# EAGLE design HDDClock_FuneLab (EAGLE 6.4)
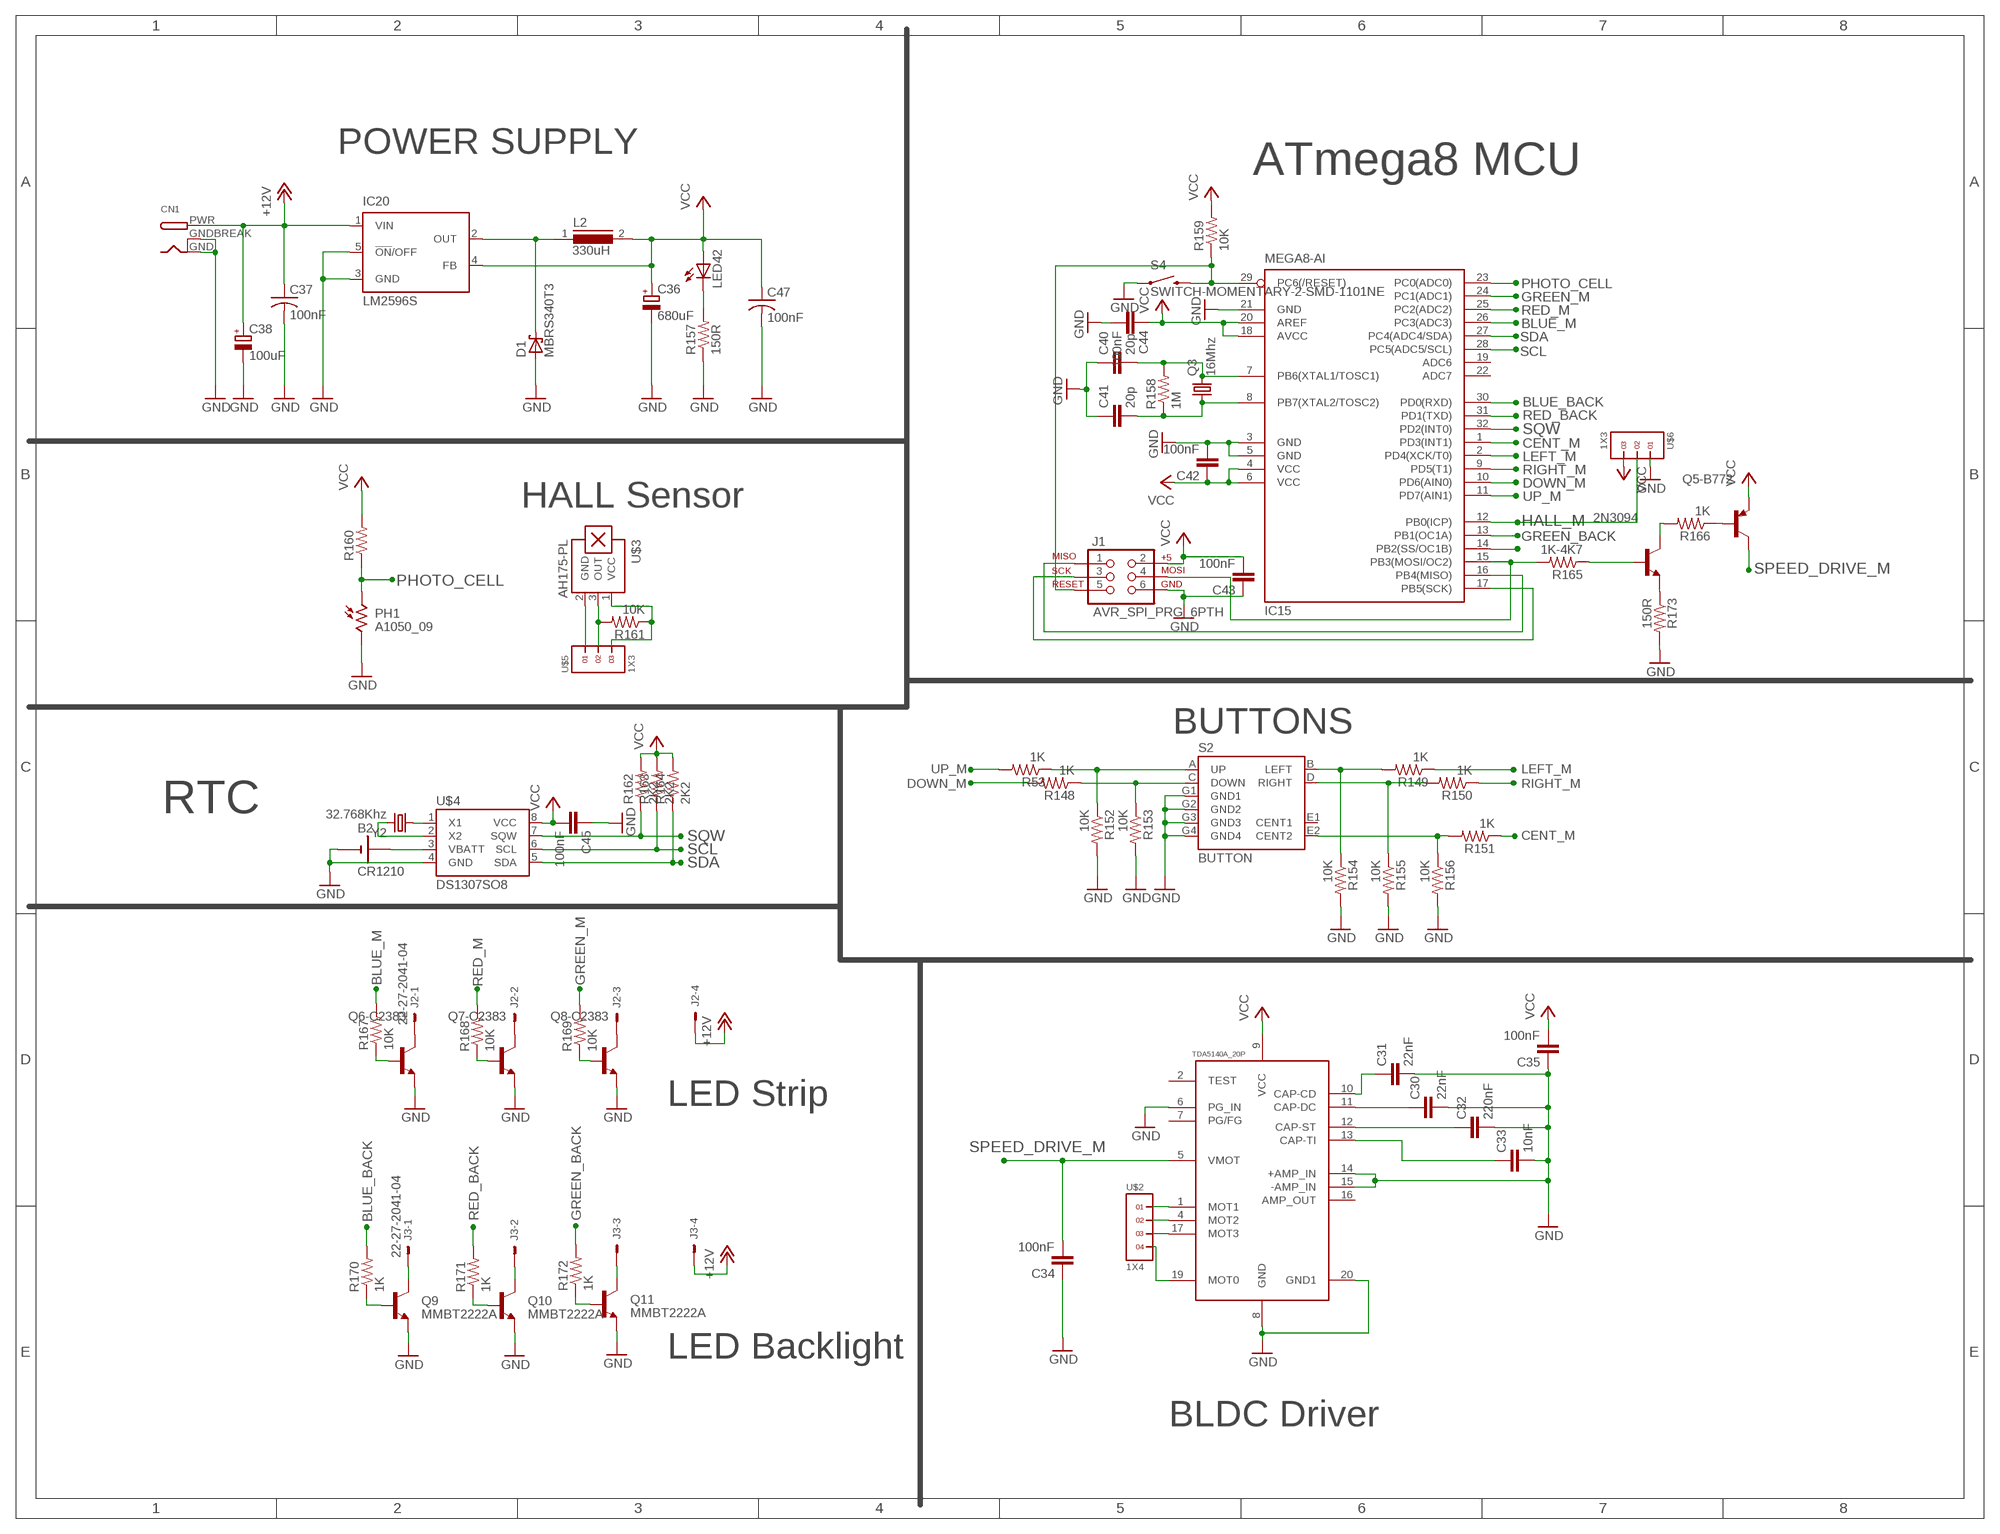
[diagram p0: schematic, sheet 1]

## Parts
2N3094  MMBT3904LT1-NPN-SOT23-BEC  [SOT23-BEC]
B2  CR1210  [CR1220_SMD]
C30  22nF  C-EUC0805K  [C0805K]
C31  22nF  C-EUC0805K  [C0805K]
C32  220nF  C-EUC0805K  [C0805K]
C33  10nF  C-EUC0805K  [C0805K]
C34  100nF  C5/2.5  [C5B2.5]
C35  100nF  C-EUC0603  [C0603]
C36  680uF  CPOL-EU153CLV-1012  [153CLV-1012]
C37  100nF  C-USC0805K  [C0805K]
C38  100uF  CPOL-EU153CLV-0605  [153CLV-0605]
C40  20p  C-EUC0603K  [C0603K]
C41  20p  C-EUC0603K  [C0603K]
C42  100nF  C-EUC0603K  [C0603K]
C43  100nF  C-EUC0603K  [C0603K]
C44  100nF  C-EUC0603K  [C0603K]
C45  100nF  C-EUC0603  [C0603]
C47  100nF  C-USC0805K  [C0805K]
CN1  DCBARRELPTH  [DCJACK_2MM_PTH]
D1  MBRS340T3  [SMC]
IC15  MEGA8-AI  [TQFP32-08]
IC20  LM2596S  [TO263-5]
J1  AVR_SPI_PRG_6PTH  [2X3]
J2  22-27-2041-04  [6410-04]
J3  22-27-2041-04  [6410-04]
L2  330uH  DR127  [DR127]
LED42  LEDCHIP-LED0805  [CHIP-LED0805]
PH1  A1050_09  [T0-46-A10XX]
Q3  16Mhz  CRYSTALHC49UP  [HC49UP]
Q5-B772  -PNP-TO126  [TO126]
Q6-C2383  -NPN-TO92-ECB  [TO92-ECB]
Q7-C2383  -NPN-TO92-ECB  [TO92-ECB]
Q8-C2383  -NPN-TO92-ECB  [TO92-ECB]
Q9  MMBT2222A  TRANSISTOR_NPNMMBT2222A  [SOT23]
Q10  MMBT2222A  TRANSISTOR_NPNMMBT2222A  [SOT23]
Q11  MMBT2222A  TRANSISTOR_NPNMMBT2222A  [SOT23]
R53  1K  R-US_R0603  [R0603]
R148  1K  R-US_R0603  [R0603]
R149  1K  R-US_R0603  [R0603]
R150  1K  R-US_R0603  [R0603]
R151  1K  R-US_R0603  [R0603]
R152  10K  R-US_R0603  [R0603]
R153  10K  R-US_R0603  [R0603]
R154  10K  R-US_R0603  [R0603]
R155  10K  R-US_R0603  [R0603]
R156  10K  R-US_R0603  [R0603]
R157  150R  R-US_R0603  [R0603]
R158  1M  R-US_R0603  [R0603]
R159  10K  R-US_R0603  [R0603]
R160  R-US_M0805  [M0805]
R161  10K  R-US_R0603  [R0603]
R162  2K2  R-US_R0603  [R0603]
R163  2K2  R-US_R0603  [R0603]
R164  2K2  R-US_R0603  [R0603]
R165  1K-4K7  R-US_R0603  [R0603]
R166  1K  R-US_R0603  [R0603]
R167  10K  R-US_R0603  [R0603]
R168  10K  R-US_R0603  [R0603]
R169  10K  R-US_R0603  [R0603]
R170  1K  R-US_R0603  [R0603]
R171  1K  R-US_R0603  [R0603]
R172  1K  R-US_R0603  [R0603]
R173  150R  R-US_R0603  [R0603]
S2  BUTTON  [BUTTON]
S4  SWITCH-MOMENTARY-2-SMD-1101NE  [TACTILE-SWITCH-1101NE]
U1  TDA5140AT_20P  [TDA5140A_20P]
U$2  1X4  [1X4]
U$3  AH175-PL  [SIP(3)]
U$4  DS1307SO8  [SO08]
U$5  1X3  [1X3]
U$6  1X3  [1X3]
Y2  32.768Khz  CRYSTAL32-SMD  [CRYSTAL-32KHZ-SMD]

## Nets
+12V: C37.1 C38.+ CN1.PWR IC20.1(VIN) J2.4 J3.4
BLUE_BACK: IC15.30(PD0(RXD)) R170.2
BLUE_M: IC15.26(PC3(ADC3)) R167.2
CENT_M: IC15.1(PD3(INT1)) R151.1
DOWN_M: IC15.10(PD6(AIN0)) R148.2
GND: B2.GND(-) C30.2 C31.2 C32.2 C33.2 C34.1 C35.1 C36.- C37.2 C38.- C40.1 C41.1 C42.2 C43.1 C44.2 C45.1 C47.2 CN1.GND CN1.GNDBREAK D1.A IC15.3(GND) IC15.5(GND) IC15.21(GND) IC20.3(GND) IC20.5(!ON!/OFF) J1.6 PH1.2 Q6-C2383.E Q7-C2383.E Q8-C2383.E Q9.2(E) Q10.2(E) Q11.2(E) R152.2 R153.2 R154.2 R155.2 R156.2 R157.1 R173.2 S2.G1(GND1) S2.G2(GND2) S2.G3(GND3) S2.G4(GND4) S4.P$1 U1.6(PG_IN) U1.8(GND) U1.14(+AMP_IN) U1.15(-AMP_IN) U1.20(GND1) U$4.4(GND) U$6.1
GREEN_BACK: IC15.13(PB1(OC1A)) R172.2
GREEN_M: IC15.24(PC1(ADC1)) R169.2
HALL_M: IC15.12(PB0(ICP)) U$6.2
LEFT_M: IC15.2(PD4(XCK/T0)) R149.1
N$9: U$3.2(GND) U$5.1
N$11: R161.2 U$3.3(OUT) U$5.2
N$25: U1.1(MOT1) U$2.1
N$28: U1.4(MOT2) U$2.2
N$29: U1.17(MOT3) U$2.3
N$31: R161.1 U$3.1(VCC) U$5.3
N$34: 2N3094.E R173.1
N$79: U1.19(MOT0) U$2.4
N$81: C31.1 U1.10(CAP-CD)
N$141: C30.1 U1.11(CAP-DC)
N$147: C32.1 U1.12(CAP-ST)
N$148: C33.1 U1.13(CAP-TI)
N$149: R53.1 R152.1 S2.A(UP)
N$186: R148.1 R153.1 S2.C(DOWN)
N$188: R149.2 R154.1 S2.B(LEFT)
N$189: R150.2 R155.1 S2.D(RIGHT)
N$312: R151.2 R156.1 S2.E2(CENT2)
N$435: LED42.C R157.2
N$438: IC15.15(PB3(MOSI/OC2)) J1.4 R165.2
N$439: IC15.29(PC6(/RESET)) J1.5 R159.1 S4.P$2
N$440: C40.2 IC15.7(PB6(XTAL1/TOSC1)) Q3.2 R158.2
N$441: C41.2 IC15.8(PB7(XTAL2/TOSC2)) Q3.1 R158.1
N$442: IC15.16(PB4(MISO)) J1.1
N$443: IC15.17(PB5(SCK)) J1.3
N$444: 2N3094.B R165.1
N$445: B2.+3V(+) U$4.3(VBATT)
N$446: 2N3094.C R166.2
N$447: U$4.1(X1) Y2.X1
N$448: U$4.2(X2) Y2.X2
N$449: Q5-B772.3(B) R166.1
N$450: J2.1 Q6-C2383.C
N$451: J2.2 Q7-C2383.C
N$452: D1.C IC20.2(OUT) L2.1
N$453: J2.3 Q8-C2383.C
N$457: IC15.14(PB2(SS/OC1B))
N$458: Q6-C2383.B R167.1
N$459: Q7-C2383.B R168.1
N$460: Q8-C2383.B R169.1
N$461: Q9.1(B) R170.1
N$463: Q10.1(B) R171.1
N$465: Q11.1(B) R172.1
N$468: J3.1 Q9.3(C)
N$469: J3.2 Q10.3(C)
N$470: J3.3 Q11.3(C)
PHOTO_CELL: IC15.23(PC0(ADC0)) PH1.1 R160.1
RED_BACK: IC15.31(PD1(TXD)) R171.2
RED_M: IC15.25(PC2(ADC2)) R168.2
RIGHT_M: IC15.9(PD5(T1)) R150.1
SCL: IC15.28(PC5(ADC5/SCL)) R163.1 U$4.6(SCL)
SDA: IC15.27(PC4(ADC4/SDA)) R164.1 U$4.5(SDA)
SPEED_DRIVE_M: C34.2 Q5-B772.2(C) U1.5(VMOT)
SQW: IC15.32(PD2(INT0)) R162.1 U$4.7(SQW)
UP_M: IC15.11(PD7(AIN1)) R53.2
VCC: C35.2 C36.+ C42.1 C43.2 C44.1 C45.2 C47.1 IC15.4(VCC) IC15.6(VCC) IC15.18(AVCC) IC15.20(AREF) IC20.4(FB) J1.2 L2.2 LED42.A Q5-B772.1(E) R159.2 R160.2 R162.2 R163.2 R164.2 U1.9(VCC) U$4.8(VCC) U$6.3
Unconnected: IC15.19(ADC6) IC15.22(ADC7) S2.E1(CENT1) U1.2(TEST) U1.7(PG/FG) U1.16(AMP_OUT)

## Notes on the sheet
- POWER SUPPLY
- ATmega8 MCU
- HALL Sensor
- BUTTONS
- RTC
- LED Strip
- LED Backlight
- BLDC Driver

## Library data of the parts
2N3094 Q6-C2383 Q7-C2383 Q8-C2383 = transistor:*-NPN-: NPN Transistror BF959 corrected 2008.03.06
B2 = ggaqquay:CR1210
C30-C33 C35 C40-C45 = resistor:C-EU: CAPACITOR, European symbol
C34 = capacitor-wima:C: CAPACITOR
C36 C38 = resistor:CPOL-EU: POLARIZED CAPACITOR, European symbol
C37 C47 = resistor:C-US: CAPACITOR, American symbol
CN1 = adafruit:DCBARREL: 2.0mm DC Barrel Jack DCJACK_2MM_PTH - Through Hole Jack (4UConnector: 05537)
D1 = diode:MBRS3*0T3: SCHOTTKY BARRIER RECTIFIER 3.0 AMPERES 20, 30, 40 VOLT
IC15 = atmel:MEGA8: MICROCONTROLLER 8 Kbytes FLASH, 1 kbytes SRAM, 512 bytes EEPROM, USART, 6-channel 10 bit ADC, 2-channel 8 bit ADC Pin compatible with Atmega48, ATMega88, ATMega168 Source: avr.lbr; MPN: ATMEGA8-16AU; OC_FARNELL: 9171371; OC_NEWARK: 73M8863
IC20 = national-semiconductor:LM2596: SIMPLE SWITCHER® Power Converter 150 kHz 3A Step-Down Voltage Regulator Source: http://www.national.com/ds/LM/LM2596.pdf; MF: NATIONAL SEMICONDUCTOR; MPN: LM2596S-ADJ/NOPB; OC_FARNELL: 9494367; OC_NEWARK: 41K3842
J1 = SparkFun:AVR_SPI_PRG_6: AVR ISP 6 Pin This is the reduced ISP connector for AVR programming. Common on Arduino. This footprint will take up less PCB space and can be used with a 10-pin to 6-pin adapter such as SKU: BOB-08508
J2 J3 = con-molex:22-?-04: CONNECTOR wire to board 2.54 mm (.1 inch) pitch header; OC_FARNELL: unknown; OC_NEWARK: unknown
L2 = inductors:DR127: High Power Density, High Efficiency, Shielded Inductors
LED42 = adafruit:LED: LED
PH1 = photo-elements:A10: Sensor Robust Light Sensing Applications
Q3 = adafruit:CRYSTAL: CRYSTAL; OC_FARNELL: unknown; OC_NEWARK: unknown
Q5-B772 = transistor:*-PNP-: PNP Transistror
Q9-Q11 = SparkFun-DiscreteSemi:TRANSISTOR_NPN: Generic NPN BJT MMBT2222A - TRANS-08049 (SOT-23, 1A 40V) MPSA42 - TRANS-09116 (SOT-23, 500mA 300V) MMBT5088LT1G - TRANS-11160 (SOT-23, 50 mA 30V); PROD_ID: TRANS-08049
R53 R148-R173 = resistor:R-US_: RESISTOR, American symbol
S2 = ggaqquay:BUTTON
S4 = SparkFun-Electromechanical:SWITCH-MOMENTARY-2: Various NO switches- pushbuttons, reed, etc
U1 = ggaqquay:TDA5140AT_20P
U$2 = headers(2mm):1X4
U$3 = ggaqquay:AH175-PL
U$4 = SparkFun-FreqCtrl:DS1307: I2C real-time clock with battery backup.
U$5 U$6 = headers(2mm):1X3
Y2 = SparkFun-FreqCtrl:CRYSTAL: Various standard crystals. Proven footprints. Spark Fun Electronics SKU : COM-00534

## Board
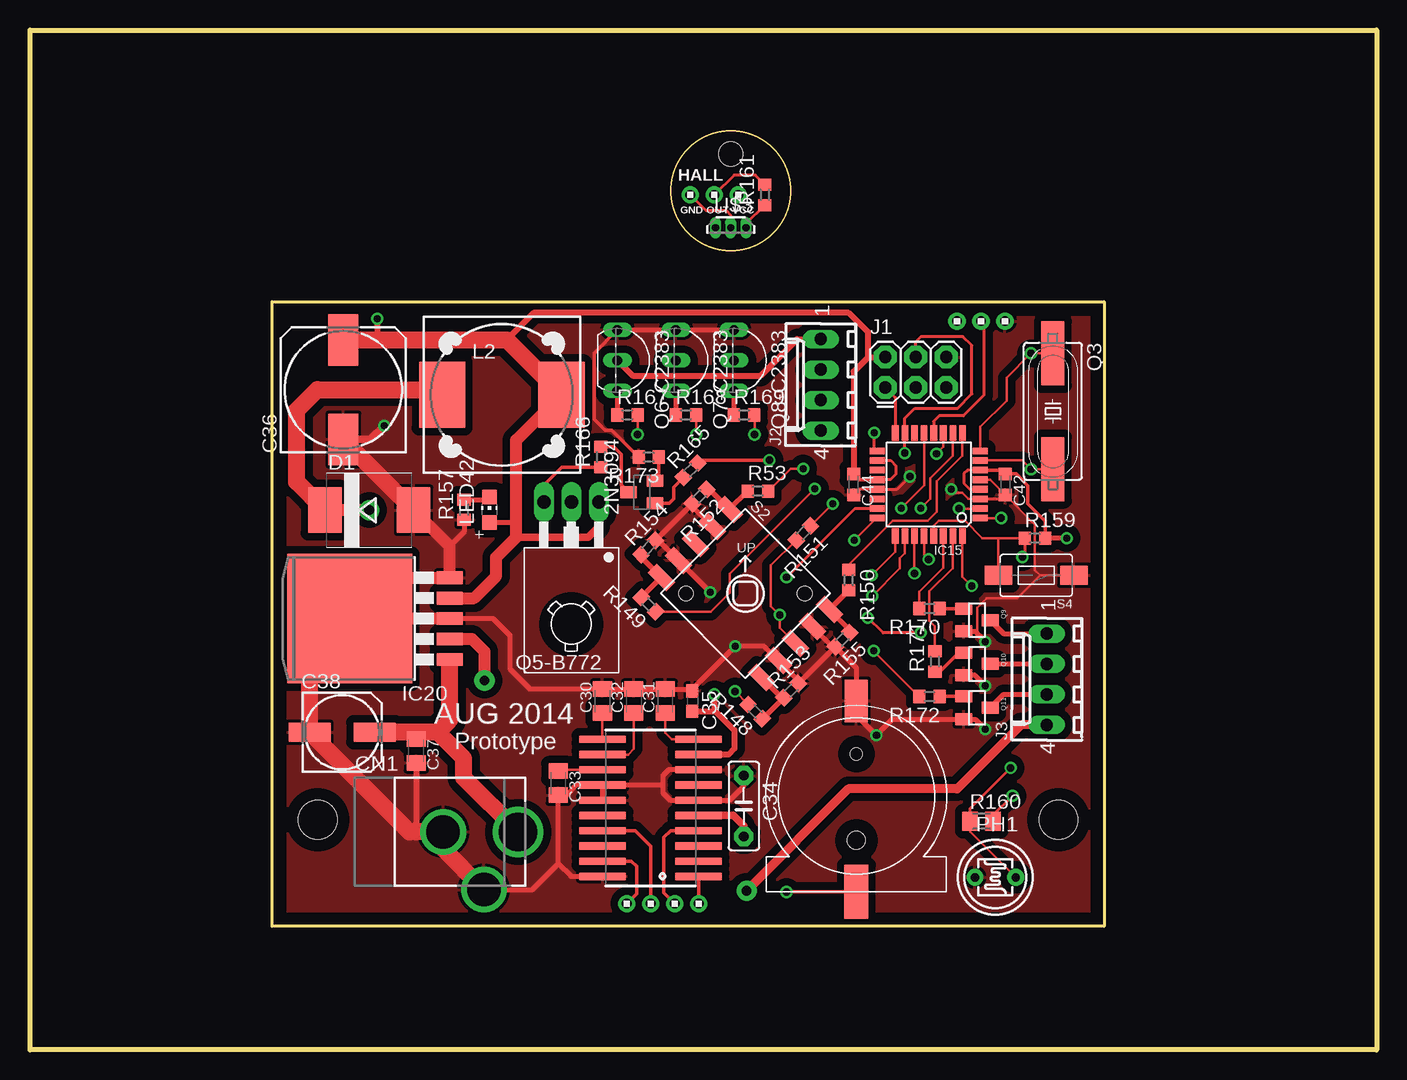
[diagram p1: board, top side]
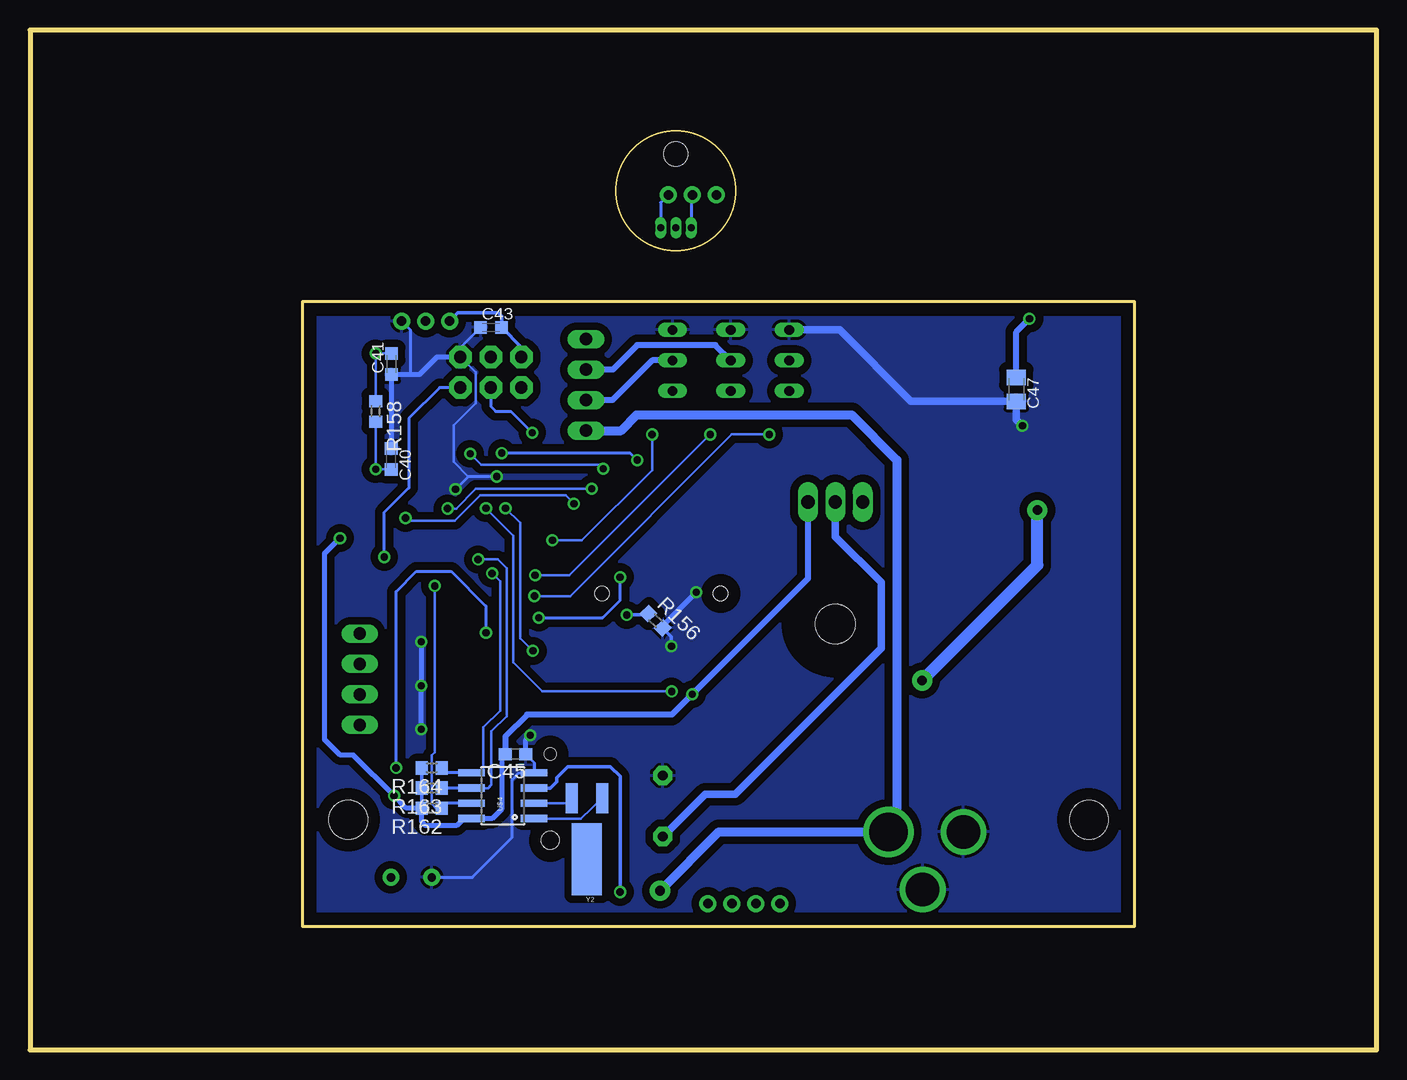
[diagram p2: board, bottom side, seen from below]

Size 112.22 x 84.99 mm. Coordinates in mm from the lower left corner, seen from the top.
Outline: 20.17,62.36 89.51,62.36 89.51,10.29 20.17,10.29 20.17,62.36
Outline: 0,0 0,84.99 112.22,84.99 112.22,0 0,0
Outline: circle at 58.39,71.6 radius 4.98
Copper layers (1*16): Top 0.035mm / dielectric 1.5mm / Bottom 0.035mm
Design rules "default *": minimum track width 10mil, minimum drill 24mil, track to track 8mil, track to pad 8mil, pad to pad 8mil, via to via 8mil, smd to smd 8mil, copper to edge 40mil, drill to drill 8mil, minimum pad ring 1mil, minimum via ring 8mil, stop-mask expansion 4mil, vias tented up to drill 0mil, thermal gap 10mil
Holes 3.2 mm at 23.98,19.18 85.7,19.18
Holes 2 mm at 58.39,74.65

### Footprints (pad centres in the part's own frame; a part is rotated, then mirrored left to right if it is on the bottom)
SOT23-BEC = smd 1 x 1.4: B -0.95,-1.1; C 0,1.1; E 0.95,-1.1
CR1220_SMD = smd 4.5 x 2: +3V 8,0 | smd 3.556 x 1.93: GND -7.919,0 | hole 1.5: 3.7,0 | hole 1: -3.5,0
C0805K = smd 1.3 x 1.6: 1 -1,0; 2 1,0
C5B2.5 = drill 0.813 pad 1.6 octagon: 1 -2.54,0; 2 2.54,0
C0603 = smd 1.1 x 1: 1 -0.85,0; 2 0.85,0
153CLV-1012 = smd 4.3 x 2.5: + 4.15,0; - -4.15,0
153CLV-0605 = smd 3.5 x 1.6: + 2.7,0; - -2.7,0
C0603K = smd 1.05 x 1.08: 1 -0.875,0; 2 0.875,0
DCJACK_2MM_PTH = drill 2.8: GND 0,7.35; GNDBREAK 4.8,10.75 | drill 3.2: PWR 0,13.6
SMC = smd 2.8 x 3.8: A 3.7,0; C -3.7,0
TQFP32-08 = smd 1.27 x 0.559: 1 -4.293,2.8; 2 -4.293,2; 3 -4.293,1.2; 4 -4.293,0.4; 5 -4.293,-0.4; 6 -4.293,-1.2; 7 -4.293,-2; 8 -4.293,-2.8; 17 4.293,-2.8; 18 4.293,-2; 19 4.293,-1.2; 20 4.293,-0.4; 21 4.293,0.4; 22 4.293,1.2; 23 4.293,2; 24 4.293,2.8 | smd 0.559 x 1.27: 9 -2.8,-4.293; 10 -2,-4.293; 11 -1.2,-4.293; 12 -0.4,-4.293; 13 0.4,-4.293; 14 1.2,-4.293; 15 2,-4.293; 16 2.8,-4.293; 25 2.8,4.293; 26 2,4.293; 27 1.2,4.293; 28 0.4,4.293; 29 -0.4,4.293; 30 -1.2,4.293; 31 -2,4.293; 32 -2.8,4.293
TO263-5 = smd 1.067 x 2.159: 1 -3.404,-5.791; 2 -1.702,-5.791; 3 0,-5.791; 4 1.702,-5.791; 5 3.404,-5.791 | smd 10.8 x 10.41: 6 0,2.54
2X3 = drill 1.016 pad 1.88 octagon: 1 0,0; 2 0,2.54; 3 2.54,0; 4 2.54,2.54; 5 5.08,0; 6 5.08,2.54
6410-04 = drill 1.016 long: 1 3.81,0; 2 1.27,0; 3 -1.27,0; 4 -3.81,0
DR127 = smd 3.85 x 5.5: 1 -4.975,0; 2 4.975,0
CHIP-LED0805 = smd 1.2 x 1.2: A 0,-1.05; C 0,1.05
T0-46-A10XX = drill 0.7 pad 1.4: 1 -1.7,0; 2 1.7,0
HC49UP = smd 5.334 x 1.93: 1 -4.826,0; 2 4.826,0
TO126 = drill 1.118 long: 1 -2.286,-5.08; 2 0,-5.08; 3 2.286,-5.08 | hole 3.302: 0,5.08
TO92-ECB = drill 0.813 long: B 2.54,0; C 0,0; E -2.54,0
SOT23 = smd 1 x 1.4: 1 -0.95,-1.1; 2 0.95,-1.1; 3 0,1.1
R0603 = smd 1 x 1.1: 1 -0.85,0; 2 0.85,0
M0805 = smd 1.3 x 1.6: 1 -0.95,0; 2 0.95,0
BUTTON = smd 2.184 x 1.067: A -5.9,4; B -5.9,-4; C 5.9,-4; D 5.9,4; E1 -5.9,0; E2 5.9,0; G1 -5.9,2; G2 -5.9,-2; G3 5.9,-2; G4 5.9,2 | hole 1.2: -3.5,-3.5; 3.5,3.5
TACTILE-SWITCH-1101NE = smd 2.3 x 1.6: P$1 -3.15,0; P$2 3.15,0
TDA5140A_20P = smd 0.6 x 3.9: 1 -5.715,-4; 2 -4.445,-4; 3 -3.175,-4; 4 -1.905,-4; 5 -0.635,-4; 6 0.635,-4; 7 1.905,-4; 8 3.175,-4; 9 4.445,-4; 10 5.715,-4; 11 5.715,4; 12 4.445,4; 13 3.175,4; 14 1.905,4; 15 0.635,4; 16 -0.635,4; 17 -1.905,4; 18 -3.175,4; 19 -4.445,4; 20 -5.715,4
1X4 = drill 0.8 pad 1.422: 1 -3,0; 2 -1,0; 3 1,0; 4 3,0
SIP(3) = drill 0.6 pad 0.7 long: 1 -1.27,0; 2 0,0; 3 1.27,0
SO08 = smd 0.61 x 2.21: 1 -1.905,-2.616; 2 -0.635,-2.616; 3 0.635,-2.616; 4 1.905,-2.616; 5 1.905,2.616; 6 0.635,2.616; 7 -0.635,2.616; 8 -1.905,2.616
1X3 = drill 0.8 pad 1.422: 1 -2,0; 2 0,0; 3 2,0
CRYSTAL-32KHZ-SMD = smd 2.5 x 6: SHEILD 0,5.08 | smd 1 x 2.5: X1 -1.27,0; X2 1.27,0

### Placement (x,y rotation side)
2N3094  50.98,46.48 90 top
B2  68.86,21.16 270 top
C30  47.7,29.06 90 top
C31  52.93,29.06 90 top
C32  50.32,29.06 90 top
C33  44.02,22.23 270 top
C34  59.49,20.32 270 top
C35  55.19,29.06 270 top
C36  26.11,55.02 90 top
C37  32.18,24.92 270 top
C38  26.01,26.47 0 top
C40  82.12,49.25 270 bottom
C41  82.09,57.15 90 bottom
C42  81.28,47.12 270 top
C43  73.79,60.2 0 bottom
C44  68.63,47.12 270 top
C45  71.75,24.64 180 bottom
C47  30.02,55.04 270 bottom
CN1  27.08,18.16 270 top
D1  28.27,44.98 0 top
IC15  74.9,47.12 180 top
IC20  29.18,35.94 90 top
J1  71.27,55.19 0 top
J2  65.89,55.42 90 top
J3  84.73,30.89 90 top
L2  39.32,54.58 0 top
LED42  38.28,45.01 0 top
PH1  80.44,14.38 180 top
Q3  85.24,53.21 270 top
Q5-B772  45.11,40.56 180 top
Q6-C2383  48.95,57.45 270 top
Q7-C2383  53.82,57.45 270 top
Q8-C2383  58.67,57.45 270 top
Q9  78.92,35.81 270 top
Q10  78.92,32.16 270 top
Q11  78.92,28.5 270 top
R53  60.66,46.56 0 top
R148  60.43,28.18 135 top
R149  51.54,37.11 135 top
R150  68.22,39.14 270 top
R151  64.44,43.07 225 top
R152  55.8,46.11 225 top
R153  63.42,29.95 45 top
R154  51.52,41.87 45 top
R155  67.7,34.19 225 top
R156  60.08,35.76 315 bottom
R157  36.17,45.01 90 top
R158  83.41,53.21 270 bottom
R159  83.74,42.65 0 top
R160  79.3,19.05 0 top
R161  61.24,71.25 90 top
R162  78.74,20.14 180 bottom
R163  78.74,21.82 180 bottom
R164  78.74,23.49 180 bottom
R165  55.05,48.31 45 top
R166  47.57,49.4 90 top
R167  49.78,52.91 0 top
R168  54.66,52.91 0 top
R169  59.51,52.91 0 top
R170  74.96,36.78 180 top
R171  75.41,32.36 90 top
R172  74.96,29.44 180 top
R173  51.56,49.4 180 top
S2  59.61,38.03 315 top
S4  83.85,39.55 180 top
U1  51.71,20.17 90 top
U$2  52.73,12.19 180 top
U$3  58.39,68.5 180 top
U$4  72.82,21.18 90 bottom
U$5  57.02,71.25 0 top
U$6  79.25,60.73 180 top
Y2  65.81,20.96 180 bottom

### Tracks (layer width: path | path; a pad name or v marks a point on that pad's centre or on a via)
+12V  (via drill 0.8 pad 1.68)
  Top 0.508: 34.98,32 IC20.1 | C37.1 32.23,25.92 32.23,26.47
  Top 0.762: v59.72,13.26 68.2,21.74 77.27,21.74 82.6,27.08 J3.4
  Top 1.422: CN1.PWR 36.14,22.69 36.14,24.28 33.96,26.47 | 33.96,26.47 32.23,26.47 C38.+ | 33.96,26.47 34.98,27.48 34.98,32
  Bottom 0.762: J2.4 62.97,51.61 61.67,52.91 43.74,52.91 39.98,49.15 39.98,18.86 CN1.PWR 54.81,18.16 v59.72,13.26
BLUE_BACK
  Top 0.203: IC15.30 76.1,40.16 74.11,38.16 R170.2
BLUE_M  (via drill 0.6)
  Top 0.203: R167.2 50.63,51.29 v50.62,51.28 | v70.18,37.82 72.49,40.13 72.49,40.97 72.9,41.38 IC15.26
  Bottom 0.203: v50.62,51.28 53.72,51.28 67.18,37.82 v70.18,37.82
CENT_M  (via drill 0.6)
  Top 0.203: IC15.1 v80.92,44.32 | R151.1 v66.89,45.52
  Bottom 0.203: v80.92,44.32 80.7,44.09 76.81,44.09 74.7,46.2 67.58,46.2 v66.89,45.52
DOWN_M  (via drill 0.6)
  Top 0.203: v58.75,29.87 R148.2 | v74.22,45.14 75.01,45.92 75.01,47.63 76.9,49.52 IC15.10
  Bottom 0.203: v74.22,45.14 71.93,42.85 71.93,32.28 69.52,29.87 v58.75,29.87
GND  (via drill 0.6)
  Top 0.203: Q10.2 77.83,31.19 | IC15.5 80.01,47.52 C42.2 83.74,43.78 83.74,39.98 84.18,39.55 | S4.P$1 84.18,39.55 | 84.18,39.55 82.27,37.64 79.73,37.64 78.92,36.83 78.92,34.7 79.03,34.58 | v76.76,46.71 77.04,46.43 77.67,46.43 78.19,45.92 IC15.3
  Top 0.254: IC15.3 80.96,45.92 C42.2 | C44.2 69.11,46.72 IC15.21 72.27,46.72 v73.33,47.78
  Top 0.305: B2.GND 68.86,28.5 | Q6-C2383.E 47.02,58.06 47.02,52.55 47.93,51.64 48.48,51.64 R173.2
  Top 0.406: R157.1 36.17,43.17 34.98,41.98 | 55.19,30.06 C31.2 C32.2 C30.2 41.7,30.06 39.98,31.78 39.98,34.57 38.61,35.94 IC20.3 | 55.19,30.06 C35.1 | U1.15 U1.14 | U1.8 53.21,23.34 52.73,22.86 52.73,22.07 | 52.73,22.07 52.73,21.41 53.34,20.8 U1.6 58.32,20.8 59.49,21.97 C34.1 | U1.14 52.73,22.07 | U1.20 45.09,14.45 44.02,15.52 | 32.18,18.9 32.18,18.19 32.21,18.16 | U1.14 45.52,22.07 44.67,21.23 C33.2 44.02,15.52 | CN1.GNDBREAK 41.86,13.36 44.02,15.52 | Q6-C2383.E Q7-C2383.E Q8-C2383.E | Q9.2 78.75,34.86 79.03,34.58 v79.6,34.01 | v79.6,30.35 78.75,31.21 Q10.2 | v79.6,26.72 78.78,27.55 Q11.2 71.87,27.55 v70.54,26.21 68.86,27.89 68.86,28.5 | S2.G1 55.2,45.27 R152.2 52.16,42.47 R154.2 52.34,42.47 S2.G2 v56.69,38.13 | S2.G4 66.89,33.58 R155.2 | B2.GND 68.86,31.82 R155.2 | R155.2 64.07,30.55 R153.2 64.02,30.79 S2.G3 61.19,33.63 v58.77,33.63 55.19,30.06
  Top 0.508: C37.2 32.18,18.9
  Top 0.61: C36.- 28.36,50.87 v29.51,52.02
  Top 1.016: D1.A 34.98,41.98 IC20.5 31.24,39.34 30.38,38.48 30.38,36.7 | IC20.3 31.14,35.94 30.38,36.7 | 26.67,36.7 30.38,36.7
  Top 1.422: CN1.GNDBREAK 34.43,16.76 CN1.GND 32.21,18.16 31.62,18.16 C38.- 23.31,33.34 26.67,36.7 | D1.A 26.11,50.84 C36.-
  Bottom 0.203: 75.69,47.78 76.91,49 76.91,52.04 75.08,53.87 75.08,56.46 J1.6
  Bottom 0.254: C45.1 70.21,23.94 U$4.4 71.48,23.09 72.03,22.53 72.03,17.7 75.36,14.38 PH1.2 | C43.1 76.35,58.51 J1.6 | U$6.1 80.54,60.03 80.54,56.28 | v73.33,47.78 75.69,47.78 v76.76,46.71
  Bottom 0.305: 70.89,24.65 C45.1 | R156.2 58.77,34.44 v58.77,33.63
  Bottom 0.406: v79.6,34.01 v79.6,30.35 v79.6,26.72 | C40.1 82.09,50.15 C41.1 80.54,56.28 79.77,56.28 78.31,57.73 J1.6 | 70.89,24.65 70.89,25.86 v70.54,26.21 | v56.69,38.13 59.48,35.33 R156.2
  Bottom 0.61: Q6-C2383.E 44.75,59.99 38.8,54.04 C47.2 30.02,52.53 v29.51,52.02
  pour Top (isolate 0.635): 20.93,10.95 88.75,10.95 88.75,61.49 20.93,61.49
  pour Bottom (isolate 0.635): 20.93,10.95 88.75,10.95 88.75,61.49 20.93,61.49
GREEN_BACK  (via drill 0.6)
  Top 0.203: v70.31,33.25 70.52,33.02 R172.2 | v72.59,45.14 74.5,47.05 IC15.13
  Bottom 0.203: v70.31,33.25 71.37,34.32 71.37,43.92 v72.59,45.14
GREEN_M  (via drill 0.6)
  Top 0.203: v68.68,42.47 70.53,44.32 IC15.24 | R169.2 60.38,52.89 v60.38,51.28
  Bottom 0.203: v60.38,51.28 60.38,48.31 66.22,42.47 v68.68,42.47
HALL_M
  Top 0.254: U$6.2 79.48,60.5 79.48,54.53 77.77,52.83 75.77,52.83 75.3,52.37 IC15.12
LEFT_M  (via drill 0.6)
  Top 0.203: R149.1 56.73,36.51 58.32,38.1 58.32,39.67 v65.41,46.76 | v77.42,45.11 IC15.2
  Bottom 0.203: v65.41,46.76 75.06,46.76 76.71,45.11 v77.42,45.11
N$9
  Top 0.254: U$5.1 56.32,69.95 58.01,69.95 58.39,69.57 U$3.2
N$11
  Top 0.254: R161.2 60.44,72.9 58.67,72.9 U$5.2
  Bottom 0.254: U$5.2 57.12,71.15 U$3.3
N$25
  Top 0.305: U1.1 55.73,14.44 U$2.1
N$28
  Top 0.305: U1.4 53.39,18.26 52.83,17.7 52.83,13.09 U$2.2
N$29
  Top 0.305: U1.17 50.42,18.26 51.73,16.95 U$2.3
N$31
  Top 0.254: R161.1 59.66,68.82 U$3.1
  Bottom 0.254: U$5.3 59.66,70.61 U$3.1
N$34
  Top 0.305: 2N3094.E 52.41,47.77 R173.1
N$79
  Top 0.305: U1.19 50.11,15.72 50.55,15.29 50.55,13.01 U$2.4
N$81
  Top 0.203: U1.10 53.49,25.88 52.93,26.44 C31.1
N$141
  Top 0.203: U1.11 47.7,25.88 C30.1
N$147
  Top 0.203: U1.12 49.83,24.61 50.32,25.1 C32.1
N$148
  Top 0.203: C33.1 44.14,23.34 U1.13
N$149
  Top 0.406: R152.1 56.59,46.71 S2.A R53.1
N$186
  Top 0.406: S2.C 62.64,29.35 R153.1 61.05,27.58 R148.1
N$188
  Top 0.406: R154.1 50.92,41.07 S2.B 52.6,39.37 R149.2
N$189
  Top 0.406: R155.1 68.3,35 S2.D R150.2
N$312  (via drill 0.6)
  Top 0.203: S2.E2 62.48,35.16 v62.48,36.25 61.75,36.98 61.75,40.37 R151.2
  Bottom 0.305: R156.1 60.8,36.25 v62.48,36.25
N$435
  Top 0.406: R157.2 38.08,45.86 LED42.C
N$438  (via drill 0.6)
  Top 0.254: v72.9,49.73 IC15.15 72.9,52.64 73.74,53.47 77.29,53.47 78.49,54.66 78.49,58.7 77.75,59.44 74.24,59.44 73.81,59 J1.4
  Top 0.305: v61.62,49.15 55.89,49.15 R165.2
  Bottom 0.254: v61.62,49.15 62.2,49.73 v72.9,49.73
N$439  (via drill 0.6)
  Top 0.203: R159.1 80.7,42.65 | 80.7,42.65 79.38,42.65 77.93,44.09 75.74,44.09 75.3,43.66 IC15.29 | S4.P$2 80.7,42.65 | 80.7,42.65
  Top 0.254: R159.1 82.91,42.63 82.91,41.28 v82.7,41.07
  Bottom 0.254: J1.5 78.08,55.19 80.65,52.63 80.65,46.84 82.7,44.78 v82.7,41.07
N$440  (via drill 0.6)
  Top 0.203: Q3.2 v83.41,48.39 82.68,49.12 IC15.7
  Bottom 0.203: C40.2 82.13,48.39 v83.41,48.39 R158.2
N$441  (via drill 0.6)
  Top 0.203: Q3.1 v83.41,58.04 81.38,56.01 81.38,54.1 79.2,51.92 IC15.8
  Bottom 0.203: C41.2 82.11,58.04 v83.41,58.04 R158.1
N$442
  Top 0.254: J1.1 72.1,54.36 IC15.16
N$443  (via drill 0.6)
  Top 0.254: IC15.17 70.36,50.17 v70.36,51.44
  Bottom 0.254: J1.3 73.81,53.62 73.41,53.21 72.14,53.21 v70.36,51.44
N$444
  Top 0.305: 2N3094.B 53.25,45.53 53.64,45.92 53.64,46.9 R165.1
N$445  (via drill 0.6)
  Top 0.305: B2.+3V v63.04,13.16
  Bottom 0.305: U$4.3 68.86,21.82 68.33,22.35 68.33,22.68 67.41,23.6 63.86,23.6 63.04,22.78 v63.04,13.16
N$446
  Top 0.305: 2N3094.C 49.28,47.08 49.28,49.63 48.65,50.25 R166.2
N$447
  Bottom 0.203: Y2.X1 66.32,19.28 U$4.1
N$448
  Bottom 0.203: Y2.X2 67.49,20.55 U$4.2
N$449
  Top 0.305: R166.1 44.31,48.55 42.82,47.07 Q5-B772.3
N$450
  Top 0.508: Q6-C2383.C 50.22,56.18 60.88,56.18 63.93,59.23 J2.1
N$451
  Bottom 0.508: Q7-C2383.C 55.09,58.72 61.62,58.72 63.65,56.69 J2.2
N$452  (via drill 0.8 pad 1.68)
  Top 1.016: v28.27,44.98 D1.C | IC20.2 36.83,34.24 37.87,33.2 v37.87,30.78
  Top 1.422: D1.C 22.23,47.33 22.23,53.29 23.95,55.02 33.91,55.02 L2.1
  Bottom 1.016: v37.87,30.78 28.27,40.39 v28.27,44.98
N$453
  Bottom 0.508: Q8-C2383.C 60.38,57.45 63.68,54.15 J2.3
N$458
  Top 0.406: Q6-C2383.B 48.93,54.9 R167.1
N$459
  Top 0.406: Q7-C2383.B R168.1
N$460
  Top 0.406: Q8-C2383.B 58.66,54.9 R169.1
N$461
  Top 0.305: R170.1 75.81,36.76 Q9.1
N$463
  Top 0.305: R171.1 75.81,31.51 77.4,33.11 Q10.1
N$465
  Top 0.305: R172.1 Q11.1
N$468
  Top 0.406: Q9.3 81.14,34.7 J3.1
N$469
  Top 0.406: Q10.3 J3.2
N$470
  Top 0.406: Q11.3 81.14,29.62 J3.3
PHOTO_CELL  (via drill 0.6)
  Top 0.203: PH1.1 78.35,18.17 R160.1
  Top 0.254: R160.1 78.35,20.13 v81.71,23.5 | v74.22,34.75 71.09,34.75 v69.82,36.02 | IC15.23 68.76,45.12 v63.04,39.4
  Bottom 0.254: v81.71,23.5 81.71,38.18 80.01,39.88 77.11,39.88 74.22,36.98 v74.22,34.75 | v69.82,36.02 64.49,36.02 63.04,37.47 v63.04,39.4
RED_BACK
  Top 0.203: IC15.31 76.9,40.15 74.96,38.2 74.96,35.76 75.41,35.31 R171.2
RED_M  (via drill 0.6)
  Top 0.203: R168.2 55.51,51.3 v55.52,51.28 | v70.13,39.55 72.1,41.52 IC15.25
  Bottom 0.203: v55.52,51.28 67.26,39.55 v70.13,39.55
RIGHT_M
  Top 0.203: R150.1 68.22,40.44 71.88,44.09 74.83,44.09 75.57,44.83 75.57,47.37 77.7,49.51 IC15.9
SCL  (via drill 0.6)
  Top 0.203: IC15.28 74.5,41.24 v74.88,40.87
  Bottom 0.203: v74.88,40.87 73.23,40.87 72.49,40.13 72.49,27.81 73.76,26.54 73.76,22.1 74.04,21.82 U$4.6
  Bottom 0.254: U$4.6 R163.1
SDA  (via drill 0.6)
  Top 0.203: IC15.27 v73.7,39.71 v73.71,39.7
  Bottom 0.203: U$4.5 74.57,23.09 74.45,23.22 74.45,26.87 73.05,28.27 73.05,39.04 v73.71,39.7
  Bottom 0.254: U$4.5 77.48,23.09 R164.1
SPEED_DRIVE_M
  Top 0.61: U1.5 58.62,19.53 59.49,18.67 C34.2
  Bottom 0.61: C34.2 55.96,21.31 53.44,21.31 41.3,33.45 41.3,38.96 45.11,42.77 Q5-B772.2
SQW  (via drill 0.6)
  Top 0.203: IC15.32 77.7,39.44 v78.49,38.66
  Bottom 0.203: v78.49,38.66 78.49,24.82 78.74,24.56 78.74,20.5 78.38,20.14 R162.1
  Bottom 0.254: U$4.7 77.48,20.55 R162.1
UP_M  (via drill 0.6)
  Top 0.203: IC15.11 76.1,50.25 v75.54,49.68 | R53.2 63.38,48.44 v64.44,48.44
  Bottom 0.203: v75.54,49.68 74.63,48.77 64.77,48.77 v64.44,48.44
VCC  (via drill 0.6)
  Top 0.203: R160.2 80.25,19.54
  Top 0.254: IC15.18 71.71,49.12 72.14,48.69 72.14,47.96 71.7,47.52 IC15.20 | IC15.6 78.11,48.32 77.83,48.03 77.83,47.22 78.33,46.72 IC15.4 | 80.25,19.54 v81.88,21.17
  Top 0.305: IC15.20 69.11,47.52 C44.1 | IC15.6 80.96,48.32 C42.1 82.18,47.99 83.16,47.02 83.16,45.49 84.59,44.06 R159.2
  Top 0.406: LED42.A 40.5,43.96 40.51,43.97 | v86.39,42.65 R159.2
  Top 0.508: v28.93,60.93 28.93,59.34 28.75,59.17 | 69.85,57.73 69.85,59.79 68.22,61.42 41.96,61.42 39.71,59.17 | 69.85,57.73 J1.2 | 69.85,57.73 68.63,56.52 C44.1 | v57.04,29.63 57.04,28.31 | 57.04,28.31 58.7,26.64 58.7,25.1 58.22,24.61 U1.9 | C35.2 56.94,28.21 57.04,28.31
  Top 0.61: 40.51,42.72 46.51,42.72 47.4,43.61 Q5-B772.1
  Top 1.016: IC20.4 37.01,37.64 38.84,39.47 38.84,41.05 40.51,42.72 40.51,43.97 40.51,50.8 L2.2
  Top 1.422: C36.+ 28.75,59.17 39.71,59.17 L2.2
  Bottom 0.305: R164.2 R163.2 R162.2 | J1.2 71.27,58.56 C43.2 72.91,61.15 73.18,61.42 76.56,61.42 U$6.3
  Bottom 0.406: v86.39,42.65 87.66,41.38 87.66,25.86 86.36,24.56 85.27,24.56 v81.88,21.17 80.85,20.14 R162.2 79.59,19.04 79.25,18.69 76.66,18.69 76.07,19.28 U$4.8 73.71,19.28 72.92,20.07 72.92,24.32 C45.2
  Bottom 0.508: C47.1 30.02,59.84 v28.93,60.93 | Q5-B772.1 47.4,39.27 v57.04,29.63 58.72,27.94 70.79,27.94 72.61,26.12 C45.2

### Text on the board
tPlace: HALL | GND OUT VCC | AUG 2014 | Prototype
